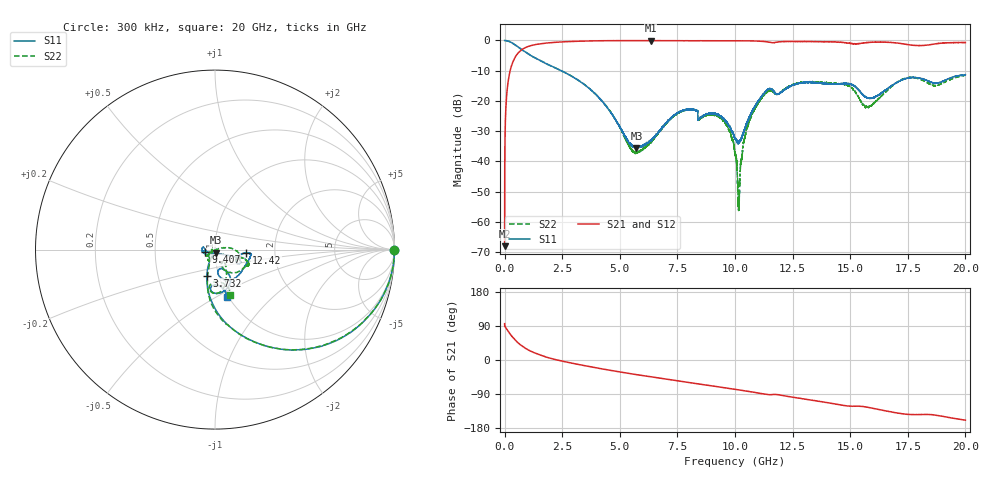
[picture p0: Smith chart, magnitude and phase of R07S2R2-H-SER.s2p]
!{R07S2R2}
!Johanson Technology Inc.
!www.johansontechnology.com
!Test Board Conditions:
!Substrate Type  RO4350B
!Substrate Thickness  10 mil
!Substrate Dk  3.66
!TL Type: GCPW
!TL Trace Width  21 mil
!TL Gap  20 mil
!Electrode orientation  Horizontal
!DUT TOPOLOGY	SERIES
!Mounting Pad LxW  16x21 mil
! Created Sat Feb  6 11:27:47 2021
# hz S ma R 50
! 2 Port Network Data from SP1.SP block
! freq  magS11  angS11  magS21  angS21  magS12  angS12  magS22  angS22
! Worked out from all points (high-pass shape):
!   20001 points, 300 kHz to 20 GHz, reference 50 ohm
!   highest |S21| = -0.05 dB at 6.333 GHz (marker M1); lowest = -68.1 dB at 300 kHz (marker M2)
!   |S21| within 3 dB of the highest: 749.1 MHz to end of sweep
!   lowest |S11| = -35.6 dB at 5.721 GHz (marker M3), VSWR 1.03, Z = 50.3 - j1.64 ohm
!   |S11| at or under -10 dB: 2.453082 GHz to 2.45381 GHz (727.9 kHz wide, 0.0297 % of centre); 2.455 GHz to end of sweep
!   |S22| runs from -56.3 to 0.0 dB; largest |S21 - S12| = 0.014
!   S11 on the Smith chart (normalised r, x): 300 kHz: open; 3.732 GHz: 0.88, -0.26; 9.407 GHz: 0.90, -0.02; 12.42 GHz: 1.42, -0.06; 20 GHz: 0.99, -0.56
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300000  0.9989 -0.3  0.0003943 95.9  0.0003798 95.6  0.9998 -0.2
1.263e8  0.9841 -11.3  0.1729 78.5  0.1735 78.5  0.9839 -11.2
4.473e8  0.8492 -36.2  0.5199 53.4  0.5211 53.5  0.8501 -36.0
1.4053e9  0.4933 -73.3  0.8636 16.3  0.8636 16.2  0.4951 -73.5
3.3343e9  0.202 -102.5  0.9727 -13.3  0.974 -13.4  0.2032 -102.0
3.7323e9  0.1535 -107.3  0.9824 -18.0  0.9823 -17.9  0.1544 -105.5
5.7213e9  0.01667 -78.5  0.9929 -38.5  0.9936 -38.5  0.01388 -172.7
6.3333e9  0.02195 -94.9  0.9948 -44.2  0.9935 -44.3  0.02035 -174.1
6.6673e9  0.03013 -118.6  0.9918 -47.4  0.9916 -47.4  0.02908 -156.6
7.8363e9  0.07106 -172.8  0.9886 -58.0  0.9898 -58.0  0.07018 -122.0
9.4073e9  0.05518 -167.4  0.9873 -72.0  0.9885 -72.0  0.05142 -146.5
1.00003e10  0.02344 -132.0  0.9873 -77.5  0.9859 -77.4  0.01361 -146.7
1.01813e10  0.02141 -90.0  0.9876 -79.0  0.9874 -79.1  0.002639 -62.0
1.04333e10  0.03538 -45.2  0.9865 -81.5  0.9857 -81.4  0.02511 13.5
1.08313e10  0.07836 -23.7  0.9792 -85.3  0.9823 -85.2  0.06964 8.2
1.14243e10  0.1548 -24.6  0.9426 -91.3  0.9436 -91.1  0.1422 -13.4
1.24213e10  0.1747 -6.5  0.9586 -97.5  0.9628 -97.6  0.1791 -18.2
1.33343e10  0.2021 -10.8  0.9573 -106.0  0.9588 -106.2  0.2058 -25.2
1.49023e10  0.1925 -56.2  0.9026 -121.3  0.903 -121.4  0.1791 -43.4
1.57183e10  0.1129 -79.5  0.9219 -124.3  0.9209 -124.5  0.07998 -58.3
1.66673e10  0.163 -61.0  0.9331 -135.7  0.9207 -135.7  0.1563 -66.4
2e10  0.2713 -75.6  0.9249 -158.8  0.9197 -158.9  0.2658 -72.2
